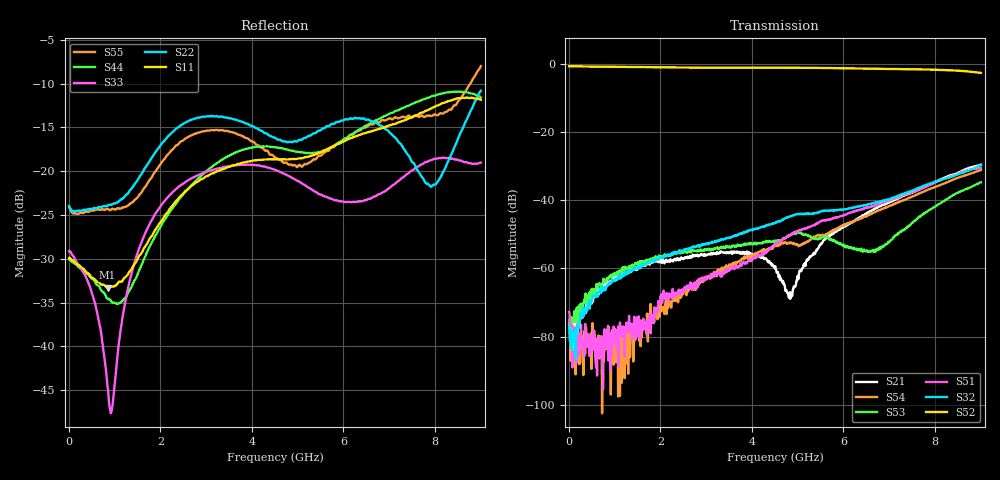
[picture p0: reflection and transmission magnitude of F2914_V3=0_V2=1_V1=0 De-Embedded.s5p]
! Integrated Device Technology
! Corporate Headquarters
! 6024 Silver Creek Valley Road
! San Jose, CA 95138  USA
! Phone:  1-408-284-8200
! Toll Free:  1-800-223-1366
! Webpage:  http://www.idt.com/
! Timing and RF Division
! 515 Groton Road, Suite 102
! Westford, MA 01886-6024
! Device:  F2914
! Description: High Reliability SP4T RF Switch
! Frequency:  0.05 -  8.GHz
! Package:  4x4 mm Thin QFN Plastic Package: 24 pin
! Ports:  5 RF,  5 DC
!  Pin  1  = GND
!  Pin  2  = GND
!  Pin  3  = GND
!  Pin  4  = GND
!  Pin  5  = RF4  =  Port 4
!  Pin  6  = GND
!  Pin  7  = GND
!  Pin  8  = RF3  =  Port 3
!  Pin  9  = GND
!  Pin 10  = GND
!  Pin 11  = RF2  =  Port 2
!  Pin 12  = GND
!  Pin 13  = GND
!  Pin 14  = RF1  =  Port 1
!  Pin 15  = GND
!  Pin 16  = Vcc
!  Pin 17  = V1
!  Pin 18  = V2
!  Pin 19  = V3
!  Pin 20  = VSSext
!  Pin 21  = GND
!  Pin 22  = RFC  =  Port 5
!  Pin 23  = GND
!  Pin 24  = GND
! Voltage:  VDD  =  +3.30 Volts
!  VSSEXT =  0.00 Volts
! Current:  IDD  = 325  uA
! State:  RF2 Selected
! V1:  Logic LOW
! V2:  Logic HIGH
! V3:  Logic LOW
! Data:  The device was measured on the F291x evaluation board which has
!  individual transmission lines to the RF pins.  Data was collected
!  using a calibrated network analyzer.  The input lines were
!  modeled using Automatic Fixture Removal (AFR) from Keysight.
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# Hz S  dB  R 50
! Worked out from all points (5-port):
!   900 points, 10 MHz to 9 GHz, reference 50 ohm
!   strongest paths, dB at 10 MHz, 2.26 GHz, 4.51 GHz, 6.76 GHz, 9 GHz:
!     S52: -0.8, -1.1, -1.2, -1.5, -2.7
!     S32: -76.5, -55.4, -46.6, -40.5, -29.8
!     S51: -72.8, -68.8, -52.9, -41.2, -30.6
!     S53: -77.1, -55.7, -51.9, -54.1, -34.8
!     S54: -76.1, -69.6, -53.4, -43.0, -31.2
!     S21: -75.8, -57.7, -59.4, -42.1, -29.6
!   lowest |S11| = -33.3 dB at 850 MHz (marker M1), VSWR 1.04, Z = 48.6 + j1.59 ohm
!   |S11| at or under -10 dB: start of sweep to end of sweep
